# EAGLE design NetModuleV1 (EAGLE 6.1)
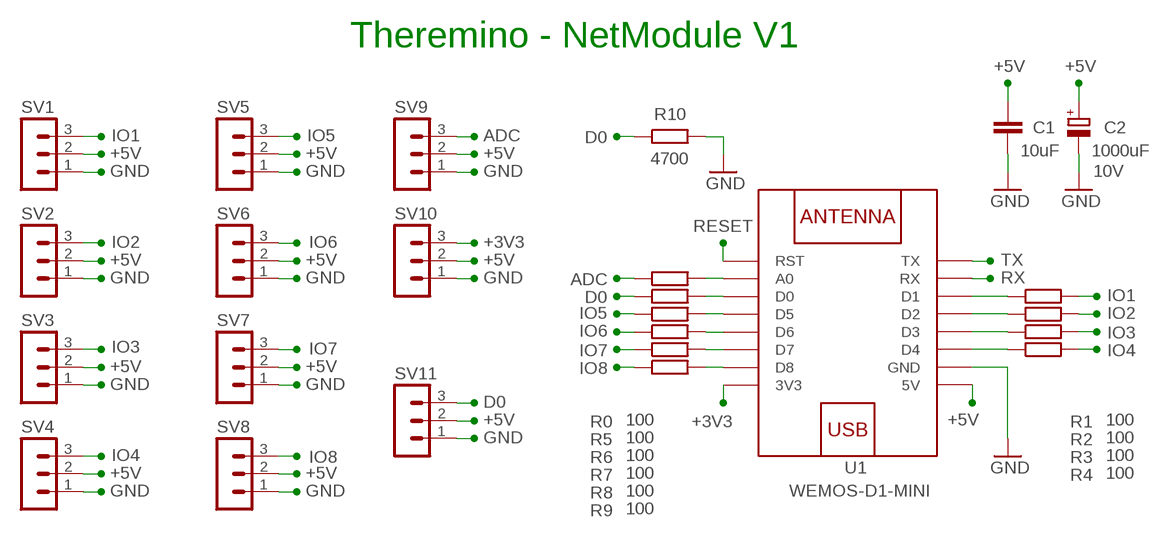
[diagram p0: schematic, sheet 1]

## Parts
C1  10uF  C-EUC0805  [C0805]
C2  1000uF  CPOL-EUE5L  [E5L]
R0  100  R-EU_R0805  [R0805]
R1  100  R-EU_R0805  [R0805]
R2  100  R-EU_R0805  [R0805]
R3  100  R-EU_R0805  [R0805]
R4  100  R-EU_R0805  [R0805]
R5  100  R-EU_R0805  [R0805]
R6  100  R-EU_R0805  [R0805]
R7  100  R-EU_R0805  [R0805]
R8  100  R-EU_R0805  [R0805]
R9  100  R-EU_R0805  [R0805]
R10  4700  R-EU_R0805  [R0805]
SV1  MA03-1L1  [MA03-1_L1]
SV2  MA03-1L1  [MA03-1_L1]
SV3  MA03-1L1  [MA03-1_L1]
SV4  MA03-1L1  [MA03-1_L1]
SV5  MA03-1L1  [MA03-1_L1]
SV6  MA03-1L1  [MA03-1_L1]
SV7  MA03-1L1  [MA03-1_L1]
SV8  MA03-1L1  [MA03-1_L1]
SV9  MA03-1L1  [MA03-1_L1]
SV10  MA03-1L1  [MA03-1_L1]
SV11  MA03-1L3  [MA03-1_L3]
U1  WEMOS-D1-MINI  [WEMOS-D1-MINI]

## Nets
+3V3: SV10.3 U1.JP1.8(3V3)
+5V: C1.1 C2.V+ SV1.2 SV2.2 SV3.2 SV4.2 SV5.2 SV6.2 SV7.2 SV8.2 SV9.2 SV10.2 SV11.2 U1.JP2.8(5V)
ADC: R9.1 SV9.3
D0: R0.1 R10.1 SV11.3
GND: C1.2 C2.V- R10.2 SV1.1 SV2.1 SV3.1 SV4.1 SV5.1 SV6.1 SV7.1 SV8.1 SV9.1 SV10.1 SV11.1 U1.JP2.7(GND)
IO1: R1.2 SV1.3
IO2: R2.2 SV2.3
IO3: R3.2 SV3.3
IO4: R4.2 SV4.3
IO5: R5.1 SV5.3
IO6: R6.1 SV6.3
IO7: R7.1 SV7.3
IO8: R8.1 SV8.3
N$1: R5.2 U1.JP1.4(D5)
N$2: R6.2 U1.JP1.5(D6)
N$3: R7.2 U1.JP1.6(D7)
N$4: R8.2 U1.JP1.7(D8)
N$5: R1.1 U1.JP2.3(D1)
N$6: R0.2 U1.JP1.3(D0)
N$7: R3.1 U1.JP2.5(D3)
N$8: R4.1 U1.JP2.6(D4)
N$9: R2.1 U1.JP2.4(D2)
N$99: R9.2 U1.JP1.2(A0)
RESET: U1.JP1.1(RST)
RX: U1.JP2.2(RX)
TX: U1.JP2.1(TX)

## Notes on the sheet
- Theremino - NetModule V1

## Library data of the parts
C1 = 00-LIVIO:C-EU: CAPACITOR, European symbol
C2 = 00-LIVIO:CPOL-EU: POLARIZED CAPACITOR, European symbol; 1: 10V
R0 R1-R10 = 00-LIVIO:R-EU_: RESISTOR, European symbol
SV1-SV11 = 03-con-lstb-M:MA03-1: PIN HEADER
U1 = 00-LIVIO:WEMOS-D1-MINI: WEMOS D1 mini: Mini Wi-Fi Board based on ESP-8266 device More details can be found here: https://www.wemos.cc/product/d1-mini.html Click here to find device on ebay.com

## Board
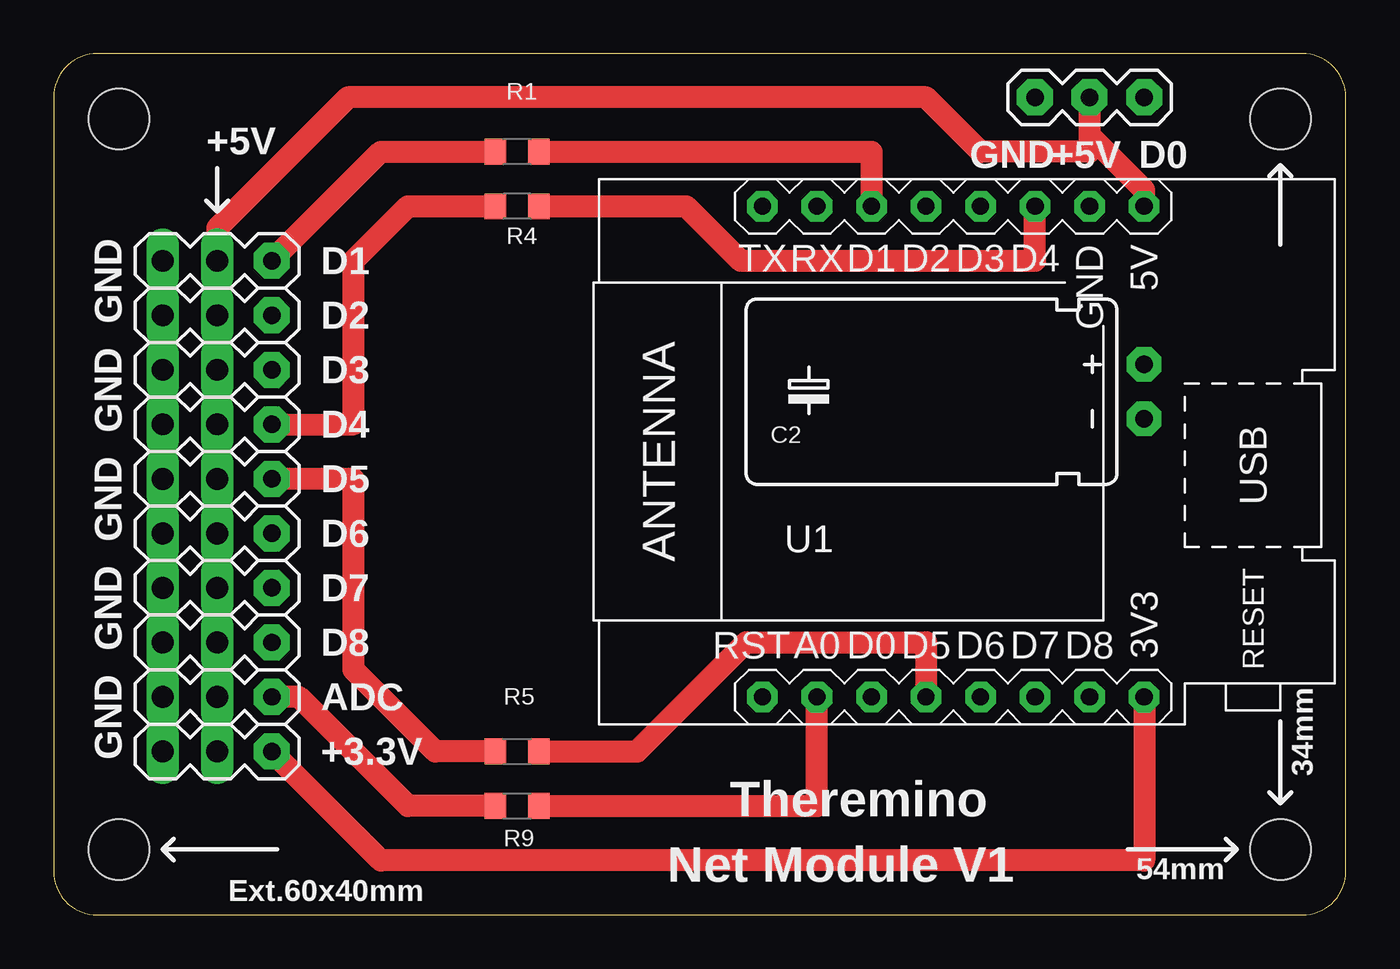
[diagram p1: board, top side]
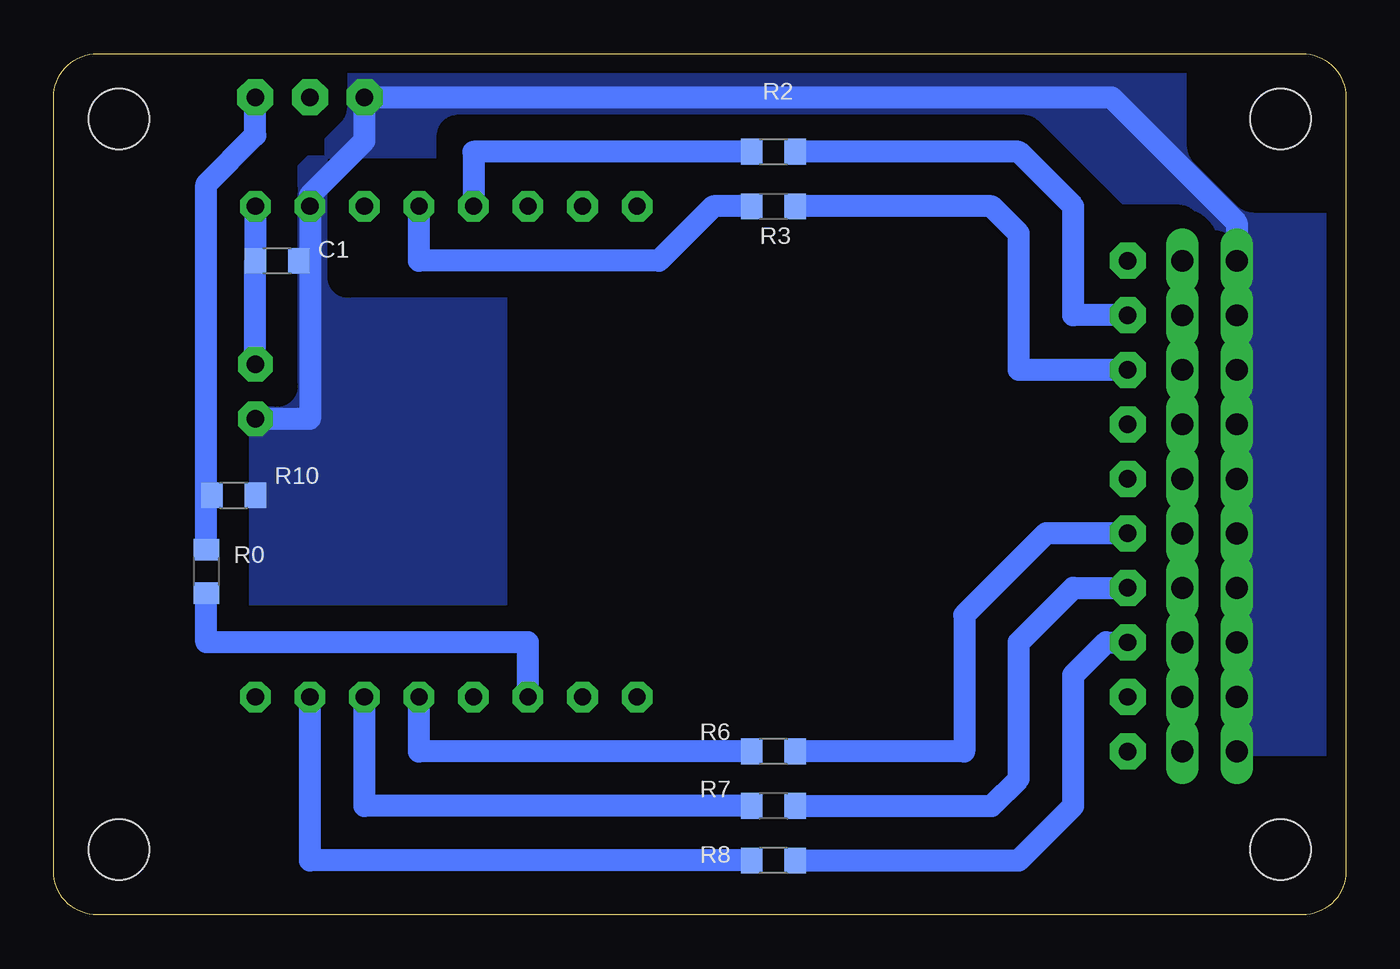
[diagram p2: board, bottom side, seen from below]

Size 60.2 x 40.13 mm. Coordinates in mm from the lower left corner, seen from the top.
Outline: 2.03,0 58.17,0 arc90 60.2,2.03 60.2,38.1 arc90 58.17,40.13 2.03,40.13 arc90 0,38.1 0,2.03 arc90 2.03,0
Copper layers (1*16): Top 0.035mm / dielectric 1.5mm / Bottom 0.035mm
Design rules: minimum track width 10mil, minimum drill 31mil, track to track 31mil, track to pad 31mil, pad to pad 31mil, via to via 31mil, smd to smd 31mil, copper to edge 31mil, drill to drill 8mil, minimum pad ring 5mil, minimum via ring 8mil, stop-mask expansion 4mil, vias tented up to drill 0mil, thermal gap 47mil
Holes 2.8 mm at 57.15,37.08 57.15,3.05 3.05,37.08 3.05,3.05
bRestrict: 29 lines

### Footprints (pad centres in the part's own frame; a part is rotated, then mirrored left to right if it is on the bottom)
C0805 = smd 1 x 1.2: 1 -1.016,0; 2 1.016,0
E5L = drill 0.813 pad 1.6 octagon: V+ -1.27,0; V- 1.27,0
R0805 = smd 1 x 1.2: 1 -1.016,0; 2 1.016,0
MA03-1_L1 = drill 1.016 long: 1 -2.54,0; 2 0,0 | drill 0.813 pad 1.676 octagon: 3 2.54,0
MA03-1_L3 = drill 0.813 pad 1.676 octagon: 1 -2.54,0; 2 0,0; 3 2.54,0
WEMOS-D1-MINI = drill 0.8 pad 1.422 octagon: JP1.1 -11.43,9.525; JP1.2 -11.43,6.985; JP1.3 -11.43,4.445; JP1.4 -11.43,1.905; JP1.5 -11.43,-0.635; JP1.6 -11.43,-3.175; JP1.7 -11.43,-5.715; JP1.8 -11.43,-8.255; JP2.1 11.43,9.525; JP2.2 11.43,6.985; JP2.3 11.43,4.445; JP2.4 11.43,1.905; JP2.5 11.43,-0.635; JP2.6 11.43,-3.175; JP2.7 11.43,-5.715; JP2.8 11.43,-8.255

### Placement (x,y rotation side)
C1  49.78,30.48 0 bottom
C2  50.8,24.38 270 top
R0  53.09,16 270 bottom
R1  21.59,35.56 180 top
R2  26.67,35.56 0 bottom
R3  26.67,33.02 0 bottom
R4  21.59,33.02 180 top
R5  21.59,7.62 0 top
R6  26.67,7.62 180 bottom
R7  26.67,5.08 180 bottom
R8  26.67,2.54 180 bottom
R9  21.59,5.08 0 top
R10  51.82,19.56 0 bottom
SV1  7.62,30.48 0 top
SV2  7.62,27.94 0 top
SV3  7.62,25.4 0 top
SV4  7.62,22.86 0 top
SV5  7.62,20.32 0 top
SV6  7.62,17.78 0 top
SV7  7.62,15.24 0 top
SV8  7.62,12.7 0 top
SV9  7.62,10.16 0 top
SV10  7.62,7.62 0 top
SV11  48.26,38.1 0 top
U1  42.55,21.59 90 top

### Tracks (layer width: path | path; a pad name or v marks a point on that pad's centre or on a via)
+3V3
  Top 1.016: U1.JP1.8 50.8,2.54 15.24,2.54 SV10.3
+5V
  Top 1.016: U1.JP2.8 50.8,33.78 48.26,36.32 | SV11.2 48.26,36.32 | 48.26,36.32 48.26,35.56 43.18,35.56 40.64,38.1 13.72,38.1 7.62,32 SV1.2
  Bottom 1.016: SV1.2 SV2.2 SV3.2 SV4.2 SV5.2 SV6.2 SV7.2 SV8.2 SV9.2 SV10.2 | U1.JP2.8 C1.1 C2.V+
ADC
  Top 1.016: R9.1 16.51,5.08 11.43,10.16 SV9.3
D0
  Bottom 1.016: R0.1 53.09,19.56 | 53.09,19.56 53.09,34.04 50.8,36.32 SV11.3 | R10.1 53.09,19.56
GND
  Bottom 1.016: SV10.1 SV9.1 SV8.1 SV7.1 SV6.1 SV5.1 SV4.1 SV3.1 SV2.1 SV1.1 5.08,32.26 10.92,38.1 SV11.1 45.72,36.07 48.26,33.53 U1.JP2.7 48.26,30.48 | 48.26,30.48 48.26,23.11 C2.V- | C1.2 48.26,30.48
  pour Bottom (isolate 0.9, rank 6, no thermals): -1,-1 61.2,-1 61.2,41.13 -1,41.13
IO1
  Top 1.016: SV1.3 15.24,35.56 R1.2
IO2
  Bottom 1.016: SV2.3 12.7,27.94 12.7,33.02 15.24,35.56 R2.2
IO3
  Bottom 1.016: SV3.3 15.24,25.4 15.24,31.75 16.51,33.02 R3.2
IO4
  Top 1.016: SV4.3 13.97,22.86 13.97,30.48 16.51,33.02 R4.2
IO5
  Top 1.016: R5.1 17.78,7.62 13.97,11.43 13.97,20.32 SV5.3
IO6
  Bottom 1.016: SV6.3 13.97,17.78 17.78,13.97 17.78,7.62 R6.1
IO7
  Bottom 1.016: R7.1 16.51,5.08 15.24,6.35 15.24,12.7 12.7,15.24 SV7.3
IO8
  Bottom 1.016: R8.1 15.24,2.54 12.7,5.08 12.7,11.18 11.18,12.7 SV8.3
N$1
  Top 1.016: R5.2 27.18,7.62 32.26,12.7 40.64,12.7 U1.JP1.4
N$2
  Bottom 1.016: R6.2 43.18,7.62 U1.JP1.5
N$3
  Bottom 1.016: R7.2 45.72,5.08 U1.JP1.6
N$4
  Bottom 1.016: R8.2 48.26,2.54 U1.JP1.7
N$5
  Top 1.016: R1.1 38.1,35.56 U1.JP2.3
N$6
  Bottom 1.016: U1.JP1.3 38.1,12.7 53.09,12.7 R0.2
N$7
  Bottom 1.016: R3.1 29.46,33.02 32,30.48 43.18,30.48 U1.JP2.5
N$8
  Top 1.016: R4.1 29.46,33.02 32,30.48 45.72,30.48 U1.JP2.6
N$9
  Bottom 1.016: R2.1 40.64,35.56 U1.JP2.4
N$99
  Top 1.016: R9.2 35.56,5.08 U1.JP1.2

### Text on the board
tNames: +5V | GND | +5V | D0 | D1 | GND | D2 | D3 | GND | D4 | D5 | GND | D6 | D7 | GND | D8 | ADC | GND | +3.3V | 34mm | Theremino | Net Module V1 | 54mm | Ext.60x40mm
